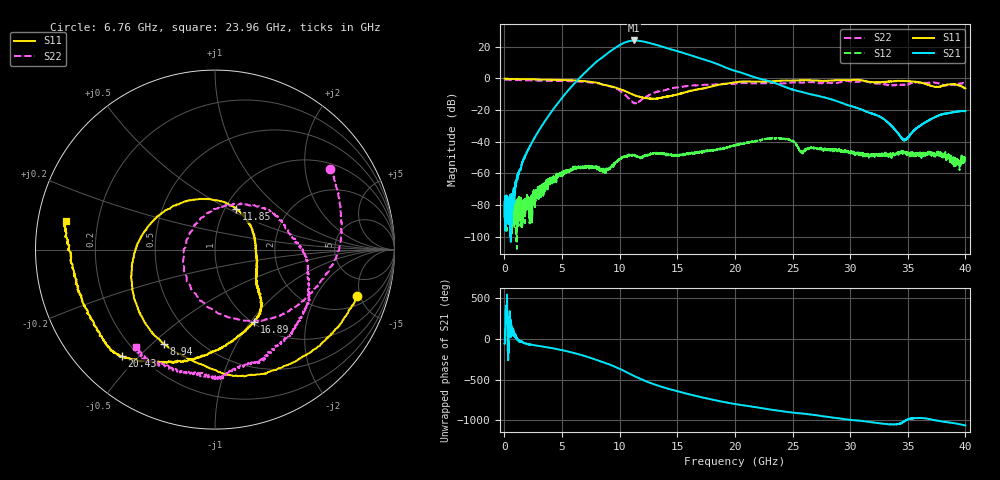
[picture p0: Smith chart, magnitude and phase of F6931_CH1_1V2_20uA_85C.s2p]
!Keysight Technologies,M9807A,MY58100526,A.15.20.05
!Date: Thursday, October 26, 2023 09:32:52
!Correction: S11(C  2-Port  )
!S21(C  2-Port  )
!S12(C  2-Port  )
!S22(C  2-Port  )
!S2P File: Measurements: S11, S21, S12, S22:
# Hz S  dB  R 50
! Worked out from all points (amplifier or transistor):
!   4000 points, 10 MHz to 40 GHz, reference 50 ohm
!   highest |S21| = 24.0 dB at 11.26 GHz (marker M1)
!   |S21| within 3 dB of that: 9.971 GHz to 13.28 GHz (3.309 GHz wide, 28.5 % of centre)
!   unconditionally stable (mu >= 1): start of sweep to end of sweep
!   at 6.67 GHz: K = 32.81, MAG = 10.7 dB, |S12| = -56.4 dB
!   at 20.01 GHz: K = 8.72, MAG = 11.3 dB, |S12| = -42.6 dB
!   at 40 GHz: K = 868.50, MAG = -16.4 dB, |S12| = -52.6 dB
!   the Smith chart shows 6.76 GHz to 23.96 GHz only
!   S11 on the Smith chart (normalised r, x): 6.76 GHz: 2.80, -4.69; 8.94 GHz: 0.33, -0.55; 11.85 GHz: 1.13, +0.54; 16.89 GHz: 1.02, -1.04; 20.43 GHz: 0.14, -0.45; 23.96 GHz: 0.08, +0.09
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1e7  -0.12 179.5  -78.01 -57.7  -83.45 -112.0  -0.73 179.7
6.68e9  -1.54 -14.9  1.44 163.9  -56.09 69.8  -2.12 37.0
6.76e9  -1.59 -18.0  2.09 160.5  -55.31 65.2  -2.13 35.2
7.95e9  -2.58 -68.4  10.32 107.0  -56.02 2.9  -3.04 5.5
8.94e9  -4.46 -118.2  15.82 56.3  -57.95 -99.6  -4.61 -24.1
9.63e9  -5.80 -153.2  19.40 16.6  -52.95 -172.0  -6.23 -52.6
1.028e10  -7.43 173.1  22.19 -25.4  -49.95 135.0  -9.23 -89.1
1.085e10  -9.22 139.1  23.62 -65.8  -48.54 102.1  -13.24 -136.8
1.126e10  -10.59 108.9  23.99 -94.9  -48.18 79.8  -15.74 171.5
1.185e10  -11.89 62.4  23.59 -133.8  -50.53 67.1  -13.67 102.3
1.251e10  -12.72 24.9  22.56 -171.6  -48.09 54.3  -10.63 60.9
1.334e10  -12.59 -10.3  20.86 146.6  -47.29 25.7  -8.32 30.7
1.412e10  -11.47 -30.4  19.08 112.8  -48.59 12.0  -7.06 7.6
1.517e10  -9.80 -42.4  16.85 71.2  -48.14 1.2  -5.45 -12.1
1.689e10  -6.77 -61.8  12.91 10.9  -47.00 -18.6  -4.28 -40.1
1.829e10  -4.49 -96.0  9.60 -33.7  -45.20 -35.3  -3.86 -59.9
2.001e10  -2.43 -125.4  4.76 -79.2  -42.65 -64.0  -3.29 -82.3
2.043e10  -2.05 -131.2  3.87 -89.2  -41.46 -73.0  -2.95 -86.6
2.396e10  -1.44 169.2  -4.24 -164.5  -37.99 174.9  -3.11 -129.0
2.667e10  -1.26 139.3  -10.20 149.7  -43.64 119.4  -2.41 -154.2
3.334e10  -1.91 11.5  -28.29 32.0  -47.54 -15.4  -4.09 114.2
4e10  -6.23 -162.2  -20.64 17.0  -52.56 -57.2  -3.00 -3.0
